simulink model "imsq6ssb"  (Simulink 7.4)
settings: Solver=ode45  StartTime=0  StopTime=0.3  MaxStep=4e-5  RelTol=1e-3  AbsTol=1e-3
undefined symbols (not defined in the file or in its folder): sgn

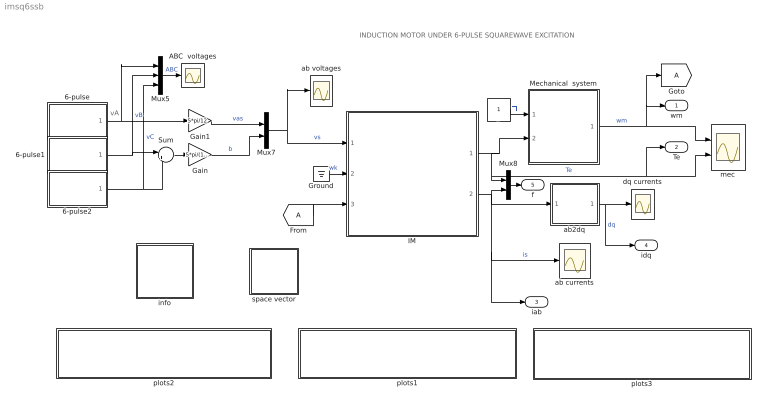
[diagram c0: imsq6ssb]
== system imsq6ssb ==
  note: vA
  note: INDUCTION MOTOR UNDER 6-PULSE SQUAREWAVE EXCITATION
  6-pulse : Subsystem  mask{A=1, w=2*pi*50, p=1e-3}
      mask prompts: A "Amplitude"; w "Frequency [rad/s]"; p "Phase [rad]"
  6-pulse1 : Subsystem  mask{A=1.0, w=2*pi*50, p=-2*pi/3+1e-3}
      mask prompts: A "Amplitude"; w "Frequency [rad/s]"; p "Phase [rad]"
  6-pulse2 : Subsystem  mask{A=1.0, w=2*pi*50, p=2*pi/3+1e-3}
      mask prompts: A "Amplitude"; w "Frequency [rad/s]"; p "Phase [rad]"
  ABC  voltages : Scope
  Gain : Gain  Gain=5*pi/(12*sqrt(3))  ParameterDataType=sfix(16)  ParameterScaling=2^0  OutDataType=sfix(16)  OutScaling=2^0
  Gain1 : Gain  Gain=5*pi/12  ParameterDataType=sfix(16)  ParameterScaling=2^0  OutDataType=sfix(16)  OutScaling=2^0
  Ground : Ground
  IM : Subsystem  mask{Rs=0.01, Rr=0.02, Lsl=0.10, Lrl=0.10, Lm=4.5, wo=2*pi*60}
      mask prompts: Rs "Stator resistance [pu]"; Rr "Rotor resistance [pu]"; Lsl "Stator leakage inductance [pu]"; Lrl "Rotor leakage inductance [pu]"; Lm "Magnetizing inductance [pu]"; wo "Base frequency [rad/s]"
  Mechanical  system : Subsystem  mask{H=0.3, Bm=1e-5}
      mask prompts: H "Inertia constant [s]"; Bm "Torque-speed coefficient"
  Mux5 : Mux  Inputs=3
  Mux7 : Mux  Inputs=2
  Mux8 : Mux  Inputs=2
  Sum : Sum  Inputs=|+-  OutDataType=sfix(16)  OutScaling=2^0
  Tl : Constant  OutDataType=sfix(16)  OutScaling=2^0
  ab currents : Scope
  ab voltages : Scope
  ab2dq : Subsystem
  dq currents : Scope
  info : Subsystem
  mec : Scope  NumInputPorts=2
  plots1 : Subsystem
  plots2 : Subsystem
  plots3 : Subsystem
  space vector : Subsystem
  wm : Outport
  Te : Outport  Port=2
  iab : Outport  Port=3
  idq : Outport  Port=4
  f : Outport  Port=5
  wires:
  Sum/1 -> Gain/1
  6-pulse1/1(Out1) -> Sum/1, Mux5/2  "vB"
  6-pulse2/1(Out1) -> Sum/2, Mux5/3  "vC"
  6-pulse/1(Out1) -> Mux5/1, Gain1/1
  Mux5/1 -> ABC  voltages/1  "ABC"
  Gain/1 -> Mux7/2  "b"
  Gain1/1 -> Mux7/1  "vas"
  Mux7/1 -> ab voltages/1, IM/1(vs)  "vs"
  Ground/1 -> IM/2(wk)  "wk"
  Tl/1 -> Mechanical  system/1(Tl)  "Tl"
  Mechanical  system/1(wm) -> mec/1, wm/1, [A]  "wm"
  IM/1(Te) -> Mechanical  system/2(Te), mec/2, Te/1, Mux8/1  "Te"
  [A] -> IM/3(wm)
  ab2dq/1(dq) -> idq/1, dq currents/1  "dq"
  Mux8/1 -> f/1
  IM/2(is) -> ab2dq/1(ab), ab currents/1, iab/1, Mux8/2  "is"

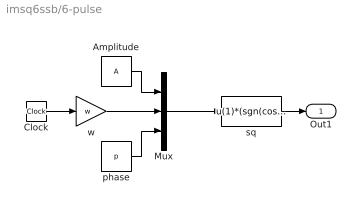
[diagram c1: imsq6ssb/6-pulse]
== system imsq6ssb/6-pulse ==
  Amplitude : Constant  Value=A  OutDataType=sfix(16)  OutScaling=2^0
  Clock : Clock
  Mux : Mux  Inputs=3
  phase : Constant  Value=p  OutDataType=sfix(16)  OutScaling=2^0
  sq : Fcn  Expr=u(1)*(sgn(cos(u(2)+u(3)))/2+sgn(cos(-3*(u(2)+u(3))))/6)
  w : Gain  Gain=w  ParameterDataType=sfix(16)  ParameterScaling=2^0  OutDataType=sfix(16)  OutScaling=2^0
  Out1 : Outport
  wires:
  Mux/1 -> sq/1
  sq/1 -> Out1/1
  Clock/1 -> w/1
  w/1 -> Mux/2
  phase/1 -> Mux/3
  Amplitude/1 -> Mux/1

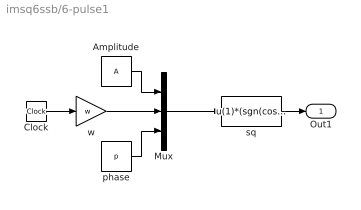
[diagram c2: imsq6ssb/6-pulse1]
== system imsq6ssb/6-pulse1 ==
  Amplitude : Constant  Value=A  OutDataType=sfix(16)  OutScaling=2^0
  Clock : Clock
  Mux : Mux  Inputs=3
  phase : Constant  Value=p  OutDataType=sfix(16)  OutScaling=2^0
  sq : Fcn  Expr=u(1)*(sgn(cos(u(2)+u(3)))/2+sgn(cos(-3*(u(2)+u(3))))/6)
  w : Gain  Gain=w  ParameterDataType=sfix(16)  ParameterScaling=2^0  OutDataType=sfix(16)  OutScaling=2^0
  Out1 : Outport
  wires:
  Amplitude/1 -> Mux/1
  phase/1 -> Mux/3
  w/1 -> Mux/2
  Clock/1 -> w/1
  sq/1 -> Out1/1
  Mux/1 -> sq/1

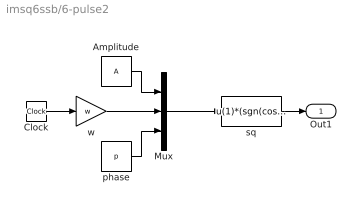
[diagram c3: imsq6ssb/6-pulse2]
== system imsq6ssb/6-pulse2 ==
  Amplitude : Constant  Value=A  OutDataType=sfix(16)  OutScaling=2^0
  Clock : Clock
  Mux : Mux  Inputs=3
  phase : Constant  Value=p  OutDataType=sfix(16)  OutScaling=2^0
  sq : Fcn  Expr=u(1)*(sgn(cos(u(2)+u(3)))/2+sgn(cos(-3*(u(2)+u(3))))/6)
  w : Gain  Gain=w  ParameterDataType=sfix(16)  ParameterScaling=2^0  OutDataType=sfix(16)  OutScaling=2^0
  Out1 : Outport
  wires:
  Mux/1 -> sq/1
  sq/1 -> Out1/1
  Clock/1 -> w/1
  w/1 -> Mux/2
  phase/1 -> Mux/3
  Amplitude/1 -> Mux/1

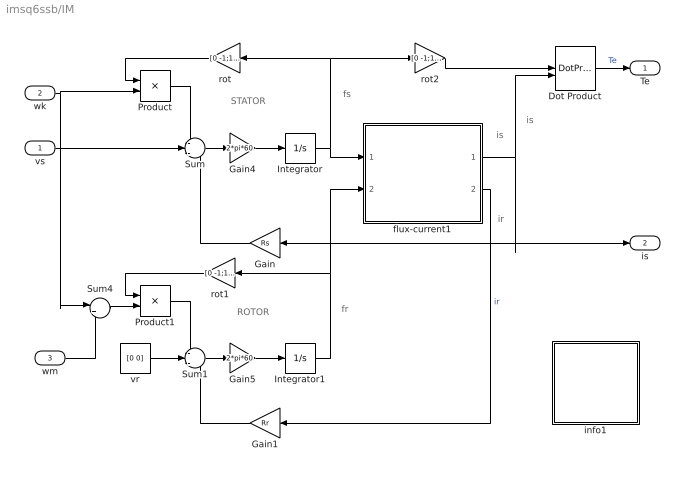
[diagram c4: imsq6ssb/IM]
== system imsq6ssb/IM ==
  note: ROTOR
  note: STATOR
  note: fs
  note: fr
  note: is
  note: is
  note: ir
  vs : Inport  OutDataType=sfix(16)  OutScaling=2^0
  wk : Inport  Port=2  OutDataType=sfix(16)  OutScaling=2^0
  wm : Inport  Port=3  OutDataType=sfix(16)  OutScaling=2^0
  Dot Product : DotProduct  OutDataType=fixdt(1, 16)  OutScaling=2^-10
  Gain : Gain  Gain=Rs  ParameterDataType=sfix(16)  ParameterScaling=2^0  OutDataType=sfix(16)  OutScaling=2^0
  Gain1 : Gain  Gain=Rr  ParameterDataType=sfix(16)  ParameterScaling=2^0  OutDataType=sfix(16)  OutScaling=2^0
  Gain4 : Gain  Gain=2*pi*60  ParameterDataType=sfix(16)  ParameterScaling=2^0  OutDataType=sfix(16)  OutScaling=2^0
  Gain5 : Gain  Gain=2*pi*60  ParameterDataType=sfix(16)  ParameterScaling=2^0  OutDataType=sfix(16)  OutScaling=2^0
  Integrator : Integrator  InitialCondition=[0 0]
  Integrator1 : Integrator  InitialCondition=[0 0]
  Product : Product  OutDataType=sfix(16)  OutScaling=2^0
  Product1 : Product  OutDataType=sfix(16)  OutScaling=2^0
  Sum : Sum  Inputs=-+-  OutDataType=sfix(16)  OutScaling=2^0
  Sum1 : Sum  Inputs=-+-  OutDataType=sfix(16)  OutScaling=2^0
  Sum4 : Sum  Inputs=|+-  OutDataType=sfix(16)  OutScaling=2^0
  flux-current1 : Subsystem
  info1 : Subsystem
  rot : Gain  Gain=[0 -1;1 0]  Multiplication=Matrix(K*u)  ParameterDataType=sfix(16)  ParameterScaling=2^0  OutDataType=sfix(16)  OutScaling=2^0
  rot1 : Gain  Gain=[0 -1;1 0]  Multiplication=Matrix(K*u)  ParameterDataType=sfix(16)  ParameterScaling=2^0  OutDataType=sfix(16)  OutScaling=2^0
  rot2 : Gain  Gain=[0 -1;1 0]  Multiplication=Matrix(K*u)  ParameterDataType=sfix(16)  ParameterScaling=2^0  OutDataType=sfix(16)  OutScaling=2^0
  vr : Constant  Value=[0 0]  OutDataType=sfix(16)  OutScaling=2^0
  Te : Outport
  is : Outport  Port=2
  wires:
  Gain/1 -> Sum/3
  vr/1 -> Sum1/2
  Gain1/1 -> Sum1/3
  flux-current1/2(ir) -> Gain1/1  "ir"
  Integrator/1 -> flux-current1/1(fs), rot/1, rot2/1
  Integrator1/1 -> flux-current1/2(fr), rot1/1
  Product1/1 -> Sum1/1
  rot1/1 -> Product1/1
  Product/1 -> Sum/1
  rot/1 -> Product/1
  rot2/1 -> Dot Product/1
  Sum4/1 -> Product1/2
  Sum/1 -> Gain4/1
  Gain4/1 -> Integrator/1
  Sum1/1 -> Gain5/1
  Gain5/1 -> Integrator1/1
  flux-current1/1(is) -> Gain/1, is/1, Dot Product/2
  Dot Product/1 -> Te/1  "Te"
  vs/1 -> Sum/2
  wk/1 -> Product/2, Sum4/1
  wm/1 -> Sum4/2

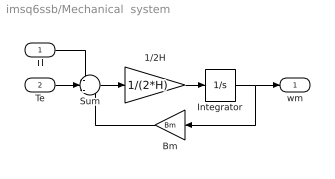
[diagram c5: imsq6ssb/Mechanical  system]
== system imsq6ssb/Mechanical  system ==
  Tl : Inport  OutDataType=sfix(16)  OutScaling=2^0
  Te : Inport  Port=2  OutDataType=sfix(16)  OutScaling=2^0
  1/2H : Gain  Gain=1/(2*H)  ParameterDataType=sfix(16)  ParameterScaling=2^0  OutDataType=sfix(16)  OutScaling=2^0
  Bm : Gain  Gain=Bm  ParameterDataType=sfix(16)  ParameterScaling=2^0  OutDataType=sfix(16)  OutScaling=2^0
  Integrator : Integrator  InitialCondition=.82
  Sum : Sum  Inputs=-+-  OutDataType=sfix(16)  OutScaling=2^0
  wm : Outport
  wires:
  Tl/1 -> Sum/1
  Te/1 -> Sum/2
  Integrator/1 -> wm/1, Bm/1
  Bm/1 -> Sum/3
  Sum/1 -> 1/2H/1
  1/2H/1 -> Integrator/1

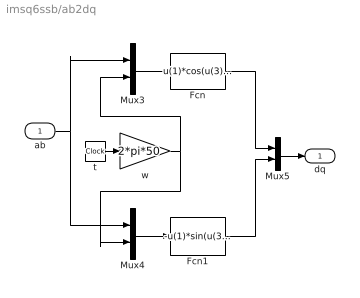
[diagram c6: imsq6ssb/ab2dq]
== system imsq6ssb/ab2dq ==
  ab : Inport  OutDataType=sfix(16)  OutScaling=2^0
  Fcn : Fcn  Expr=u(1)*cos(u(3))+u(2)*sin(u(3))
  Fcn1 : Fcn  Expr=-u(1)*sin(u(3))+u(2)*cos(u(3))
  Mux3 : Mux  Inputs=2
  Mux4 : Mux  Inputs=2
  Mux5 : Mux  Inputs=2
  t : Clock
  w : Gain  Gain=2*pi*50  ParameterDataType=sfix(16)  ParameterScaling=2^0  OutDataType=sfix(16)  OutScaling=2^0
  dq : Outport
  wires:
  t/1 -> w/1
  Mux3/1 -> Fcn/1
  Mux4/1 -> Fcn1/1
  w/1 -> Mux3/2, Mux4/2
  ab/1 -> Mux3/1, Mux4/1
  Fcn1/1 -> Mux5/2
  Fcn/1 -> Mux5/1
  Mux5/1 -> dq/1

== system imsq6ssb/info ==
  note: An induction motor under 6-pulse squarewave excitation
  note: If you modify the system parameters, follow these steps to establish the new IC state: First obtain the operating point IC's by saving to workspace the simulation parameters defined as "Final state" ic. Run the simulation for a sufficiently long enough time (~0.5s)to reach a steady-state condition. Then load from workspace the previously computed ic as "Initial state" in the Simulation parameters. Finally rerun the simulation for a specified time (in particular one cycle).

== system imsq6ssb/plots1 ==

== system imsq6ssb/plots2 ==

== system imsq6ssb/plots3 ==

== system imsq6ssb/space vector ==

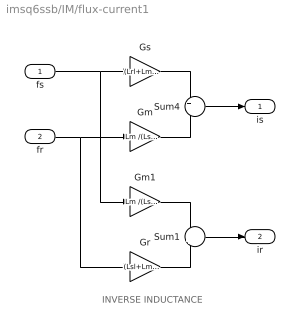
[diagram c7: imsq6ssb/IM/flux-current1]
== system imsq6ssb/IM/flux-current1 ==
  note: INVERSE INDUCTANCE
  fs : Inport  OutDataType=sfix(16)  OutScaling=2^0
  fr : Inport  Port=2  OutDataType=sfix(16)  OutScaling=2^0
  Gm : Gain  Gain=Lm /(Lsl*Lrl+Lsl*Lm+Lrl*Lm)  ParameterDataType=sfix(16)  ParameterScaling=2^0  OutDataType=sfix(16)  OutScaling=2^0
  Gm1 : Gain  Gain=Lm /(Lsl*Lrl+Lsl*Lm+Lrl*Lm)  ParameterDataType=sfix(16)  ParameterScaling=2^0  OutDataType=sfix(16)  OutScaling=2^0
  Gr : Gain  Gain=(Lsl+Lm )/(Lsl*Lrl+Lsl*Lm+Lrl*Lm)  ParameterDataType=sfix(16)  ParameterScaling=2^0  OutDataType=sfix(16)  OutScaling=2^0
  Gs : Gain  Gain=(Lrl+Lm) /(Lsl*Lrl+Lsl*Lm+Lrl*Lm)  ParameterDataType=sfix(16)  ParameterScaling=2^0  OutDataType=sfix(16)  OutScaling=2^0
  Sum1 : Sum  Inputs=-+  OutDataType=sfix(16)  OutScaling=2^0
  Sum4 : Sum  Inputs=+-  OutDataType=sfix(16)  OutScaling=2^0
  is : Outport
  ir : Outport  Port=2
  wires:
  fs/1 -> Gs/1, Gm1/1
  Gs/1 -> Sum4/1
  fr/1 -> Gm/1, Gr/1
  Gm/1 -> Sum4/2
  Sum4/1 -> is/1
  Gm1/1 -> Sum1/1
  Gr/1 -> Sum1/2
  Sum1/1 -> ir/1

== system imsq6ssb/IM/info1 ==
  note: This demonstration illustrates the dynamics of a synchronous generator, initially at no load, following a three-phase short circuit at the terminals.
  note: Synchronous machine transients under shortcircuit
